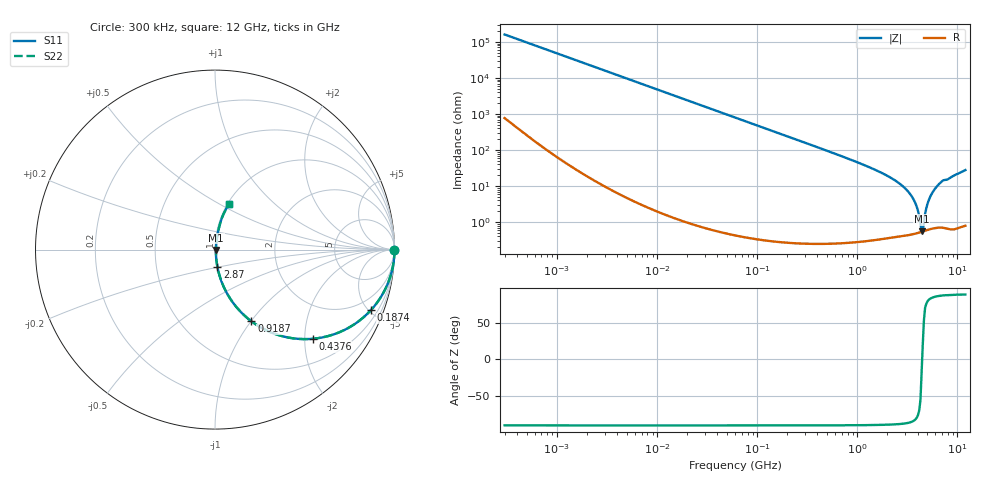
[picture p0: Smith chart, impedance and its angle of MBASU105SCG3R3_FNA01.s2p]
! MBASU105SCG3R3_FNA01  S-PARAMETER MODEL  ( Standard Model )
! Model Generated by TAIYO YUDEN Corporation (http://www.ty-top.com)
! Version 1.0
! TAIYO YUDEN Control No. 230609
! Copyright(c) 2023 TAIYO YUDEN CO.,LTD. All Rights Reserved.
! Product Description (link to TY-COMPAS)
! https://ds.yuden.co.jp/TYCOMPAS/or/detail?pn=MBASU105SCG3R3CFNA01&u=M
! Products Name : Multilayer Ceramic Capacitors
! Characteristics :
!  Capacitance : 3.3 [pF] , Rated Voltage : 50 [V] , TCC : CG / C0G
!  Case Size : 1.0 x 0.5 / 0.039 x 0.02 [mm/inch] , Thickness : 0.5 / 0.02 [mm/inch]
!  (Conditions: Temperature = 25 [degC] , DC Bias Voltage = 0 [V])
! External Node Assignments :
!  1  o---| |---o  2
! GND o---------o GND
! Frequency Range : 0.3MHz  -  12000MHz  [ 401 STEP ]
# MHZ S RI R 50
! Freq[MHz].  S11 Real  S11 Imag  S21 Real  S21 Imag  S12 Real  S12 Imag  S22 Real  S22 Imag
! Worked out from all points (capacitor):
!   401 points, 300 kHz to 12 GHz, reference 50 ohm
!   read as one part in series: C = 3.3 pF near 316.3 kHz
!   lowest |Z| = 561 mohm at 4.385 GHz (marker M1)
!   series resonance near 4.437 GHz, so ESL is about 390 pH
!   S11 on the Smith chart (normalised r, x): 300 kHz: open; 187.4 MHz: 1.01, -5.14; 437.6 MHz: 1.00, -2.18; 918.7 MHz: 1.01, -1.00; 2.87 GHz: 1.01, -0.19; 12 GHz: 1.02, +0.56
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0.3  1 -0.000622  3.37e-06 0.000622  3.37e-06 0.000622  1 -0.000622
1.769972  1 -0.00367  1.65e-05 0.00367  1.65e-05 0.00367  1 -0.00367
10.44266  0.9995 -0.0216  0.000477 0.0216  0.000477 0.0216  0.9995 -0.0216
60  0.9847 -0.1225  0.0153 0.1225  0.0153 0.1225  0.9847 -0.1225
187.4445  0.8681 -0.3379  0.1319 0.3379  0.1319 0.3379  0.8681 -0.3379
353.9943  0.6467 -0.4771  0.3533 0.4771  0.3533 0.4771  0.6467 -0.4771
437.5599  0.5435 -0.497  0.4565 0.497  0.4565 0.497  0.5435 -0.497
918.7169  0.2028 -0.3993  0.7972 0.3993  0.7972 0.3993  0.2028 -0.3993
2088.533  0.0345 -0.1725  0.9655 0.1725  0.9655 0.1725  0.0345 -0.1725
2870.14  0.0133 -0.0955  0.9867 0.0955  0.9867 0.0955  0.0133 -0.0955
3364.605  0.00799 -0.0595  0.992 0.0595  0.992 0.0595  0.00799 -0.0595
3740.715  0.00604 -0.0362  0.994 0.0362  0.994 0.0362  0.00604 -0.0362
3944.255  0.00552 -0.0246  0.9945 0.0246  0.9945 0.0246  0.00552 -0.0246
4270.516  0.00528 -0.00742  0.9947 0.00742  0.9947 0.00742  0.00528 -0.00742
4385.161  0.00535 -0.00157  0.9946 0.00157  0.9946 0.00157  0.00535 -0.00157
4502.883  0.00548 0.00199  0.9945 -0.00199  0.9945 -0.00199  0.00548 0.00199
4623.766  0.00566 0.00746  0.9943 -0.00746  0.9943 -0.00746  0.00566 0.00746
5006.236  0.00695 0.0304  0.993 -0.0304  0.993 -0.0304  0.00695 0.0304
5278.635  0.00841 0.0458  0.9916 -0.0458  0.9916 -0.0458  0.00841 0.0458
6188.031  0.0158 0.0936  0.9842 -0.0936  0.9842 -0.0936  0.0158 0.0936
7064.448  0.0255 0.1342  0.9745 -0.1342  0.9745 -0.1342  0.0255 0.1342
12000  0.0782 0.2546  0.9218 -0.2546  0.9218 -0.2546  0.0782 0.2546
